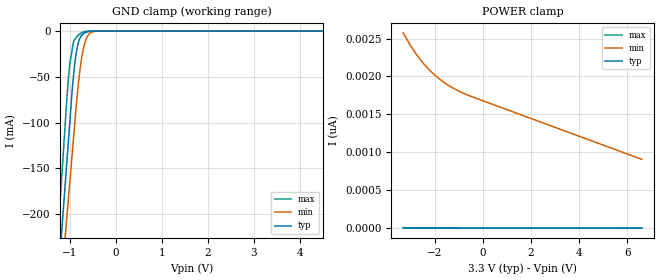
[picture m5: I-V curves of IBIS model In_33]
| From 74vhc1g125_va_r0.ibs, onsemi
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|//////////////////////////////////////////////////////////////////////////////
|//////////////////////////////////////////////////////////////////////////////
[Model]  In_33
Model_type Input
Vinh = 2.31
Vinl = 0.99
|  variable   typ   min   max
C_comp   2.7pF   2.7pF   2.7pF
|//////////////////////////////////////////////////////////////////////////////
[Temperature Range]   25   125   -55
|//////////////////////////////////////////////////////////////////////////////
[Voltage Range]   3.30V   3.00V   3.60V
|//////////////////////////////////////////////////////////////////////////////
[POWER Clamp Reference] 3.30V   3.00V   3.60V
|//////////////////////////////////////////////////////////////////////////////
[GND Clamp Reference]   0V   0V   0V
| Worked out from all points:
|   GND clamp passes 1 mA (typ) near -0.63 V on its own axis
|//////////////////////////////////////////////////////////////////////////////
[GND Clamp]
|   Voltage   I(typ)   I(min)   I(max)
-3.3V     -1.666A    -1.539A    -1.781A
-1.28V    -292mA     -334.2mA   -241.4mA
-1.22V    -251.1mA   -298.4mA   -195.7mA
-1.16V    -210.3mA   -262.7mA   -150mA
-1.08V    -155.9mA   -214.9mA   -89mA
-1V       -101.5mA   -167.2mA   -37.31mA
-920mV    -50.61mA   -119.5mA   -12.71mA
-860mV    -24.87mA   -83.72mA   -6.987mA
-720mV    -3.652mA   -23.71mA   -1.367mA
-600mV    -604.4uA   -4.518mA   -51.55uA
-420mV    -2.933uA   -150.4uA   -8.422nA
6.6V      2.301pA    2.102nA    797fA
|//////////////////////////////////////////////////////////////////////////////
[POWER Clamp]
|   Voltage   I(typ)   I(min)   I(max)
-3.3V     5.927pA    2.575nA    823.4fA
-3V       4.207pA    2.409nA    797fA
-2.8V     3.227pA    2.312nA    779.5fA
-2.6V     2.655pA    2.225nA    761.9fA
-2.4V     2.333pA    2.149nA    744.4fA
-2.2V     2.108pA    2.082nA    726.8fA
-1.8V     1.905pA    1.968nA    691.7fA
-1.6V     1.851pA    1.92nA     674.2fA
-1.2V     1.745pA    1.841nA    639.1fA
-600mV    1.586pA    1.751nA    586.4fA
6.6V      -319.7fA   907.4pA    -45.54fA
